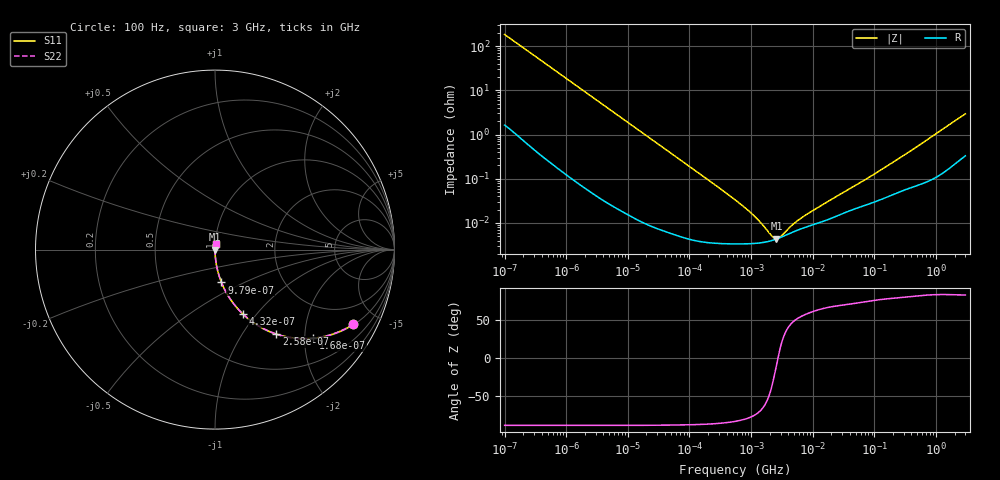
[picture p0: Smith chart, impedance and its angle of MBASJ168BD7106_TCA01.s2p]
! MBASJ168BD7106_TCA01  S-PARAMETER MODEL  ( Standard Model )
! Model Generated by TAIYO YUDEN Corporation (http://www.ty-top.com)
! Version 2.0
! TAIYO YUDEN Control No. 240328
! Copyright(c) 2022 TAIYO YUDEN CO.,LTD. All Rights Reserved.
! Product Description (link to TY-COMPAS)
! https://ds.yuden.co.jp/TYCOMPAS/or/detail?pn=MBASJ168BD7106MTCA01&u=M
! Products Name : Multilayer Ceramic Capacitors
! Characteristics :
!  Capacitance : 10 [uF] , Rated Voltage : 6.3 [V] , TCC : X7T
!  Case Size : 1.6 x 0.8 / 0.063 x 0.031 [mm/inch] , Thickness : 0.8 / 0.031 [mm/inch]
!  (Conditions: Temperature = 25 [degC] , DC Bias Voltage = 0 [V])
! External Node Assignments :
!  1  o---| |---o  2
! GND o---------o GND
! Frequency Range : 100Hz  -  3GHz  [ 401 STEP ]
# MHZ S RI R 50
! Freq[MHz].  S11 Real  S11 Imag  S21 Real  S21 Imag  S12 Real  S12 Imag  S22 Real  S22 Imag
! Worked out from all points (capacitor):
!   401 points, 100 Hz to 3 GHz, reference 50 ohm
!   read as one part in series: C = 8.62 uF near 109 Hz
!   lowest |Z| = 4.39 mohm at 2.579 MHz (marker M1)
!   series resonance near 2.725 MHz, so ESL is about 400 pH
!   S11 on the Smith chart (normalised r, x): 100 Hz: 1.03, -3.68; 168 Hz: 1.02, -2.21; 258 Hz: 1.01, -1.44; 432 Hz: 1.01, -0.86; 979 Hz: 1.00, -0.38; 3 GHz: 1.01, +0.06
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0.0001  0.7704 -0.4162  0.2296 0.4162  0.2296 0.4162  0.7704 -0.4162
0.000119  0.7052 -0.4516  0.2948 0.4516  0.2948 0.4516  0.7052 -0.4516
0.000168  0.5484 -0.4935  0.4516 0.4935  0.4516 0.4935  0.5484 -0.4935
0.000258  0.3417 -0.4705  0.6583 0.4705  0.6583 0.4705  0.3417 -0.4705
0.000348  0.2225 -0.4124  0.7775 0.4124  0.7775 0.4124  0.2225 -0.4124
0.000432  0.1576 -0.3609  0.8424 0.3609  0.8424 0.3609  0.1576 -0.3609
0.000636  0.0802 -0.2682  0.9198 0.2682  0.9198 0.2682  0.0802 -0.2682
0.000979  0.0361 -0.1832  0.9639 0.1832  0.9639 0.1832  0.0361 -0.1832
0.001788  0.0114 -0.1031  0.9886 0.1031  0.9886 0.1031  0.0114 -0.1031
0.005476  0.00142 -0.0342  0.9986 0.0342  0.9986 0.0342  0.00142 -0.0342
0.031977  0.000107 -0.0059  0.9999 0.0059  0.9999 0.0059  0.000107 -0.0059
0.547723  3.36e-05 -0.000333  1 0.000333  1 0.000333  3.36e-05 -0.000333
0.87939  3.37e-05 -0.000193  1 0.000193  1 0.000193  3.37e-05 -0.000193
1.411895  3.53e-05 -9.75e-05  1 9.75e-05  1 9.75e-05  3.53e-05 -9.75e-05
1.6065  3.63e-05 -7.6e-05  1 7.6e-05  1 7.6e-05  3.63e-05 -7.6e-05
2.579298  4.33e-05 -7.22e-06  1 7.22e-06  1 7.22e-06  4.33e-05 -7.22e-06
4.91919  6.32e-05 7.23e-05  0.9999 -7.23e-05  0.9999 -7.23e-05  6.32e-05 7.23e-05
5.361412  6.64e-05 8.25e-05  0.9999 -8.25e-05  0.9999 -8.25e-05  6.64e-05 8.25e-05
9.794414  8.95e-05 0.000164  0.9999 -0.000164  0.9999 -0.000164  8.95e-05 0.000164
67.94454  0.000246 0.000884  0.9998 -0.000884  0.9998 -0.000884  0.000246 0.000884
175.1444  0.000409 0.00205  0.9996 -0.00205  0.9996 -0.00205  0.000409 0.00205
3000  0.00413 0.029  0.9959 -0.029  0.9959 -0.029  0.00413 0.029
